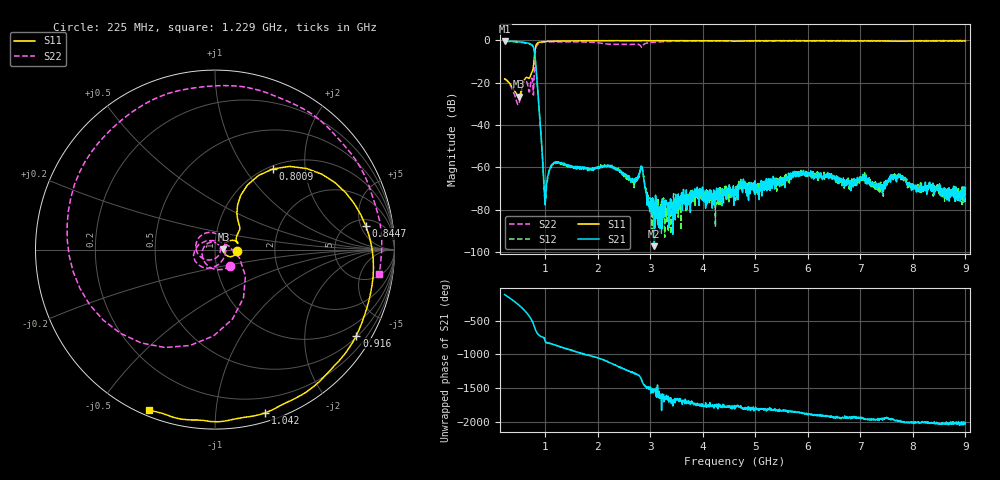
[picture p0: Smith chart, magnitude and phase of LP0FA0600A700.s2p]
!Agilent Technologies,E8358A,US41080443,A.07.50.56
!Agilent E8358A: A.07.50.56
!Date: Wednesday, August 31, 2016 09:10:34
!Correction: S11(Full 2 Port(1,2))
!S21(Full 2 Port(1,2))
!S12(Full 2 Port(1,2))
!S22(Full 2 Port(1,2))
!S2P File: Measurements: S11, S21, S12, S22:
# Hz S  dB  R 50
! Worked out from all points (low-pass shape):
!   1601 points, 225 MHz to 9 GHz, reference 50 ohm
!   highest |S21| = -0.28 dB at 225 MHz (marker M1); lowest = -97.2 dB at 3.077 GHz (marker M2)
!   |S21| within 3 dB of the highest: start of sweep to 776.3 MHz
!   lowest |S11| = -26.6 dB at 493.7 MHz (marker M3), VSWR 1.10, Z = 54.9 + j0.169 ohm
!   |S11| at or under -10 dB: start of sweep to 782.7 MHz
!   |S22| runs from -30.4 to 0.0 dB; largest |S21 - S12| = 0.021
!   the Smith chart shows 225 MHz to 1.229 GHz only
!   S11 on the Smith chart (normalised r, x): 225 MHz: 1.28, -0.01; 800.9 MHz: 1.05, +1.36; 844.7 MHz: 6.40, +6.14; 916 MHz: 0.55, -3.49; 1.042 GHz: 0.07, -1.35; 1.229 GHz: 0.02, -0.67
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2.25e8  -18.27 -2.7  -0.28 -113.7  -0.46 -113.4  -18.14 -47.5
4.937344e8  -26.58 1.9  -0.58 92.1  -0.77 92.4  -30.23 -12.7
6.034219e8  -18.56 25.7  -0.92 12.0  -1.10 12.2  -19.40 175.0
6.911719e8  -17.88 21.4  -1.39 -70.1  -1.57 -69.8  -24.24 13.4
8.008594e8  -5.14 54.3  -6.65 110.5  -6.84 110.7  -7.96 -76.0
8.447344e8  -1.41 9.0  -19.79 36.9  -19.95 36.9  -2.12 -164.1
9.160312e8  -0.71 -31.3  -43.67 -13.3  -43.90 -13.4  -1.05 130.2
1.042172e9  -0.44 -72.9  -64.58 -111.3  -66.06 -104.8  -0.72 64.6
1.228641e9  -0.30 -112.5  -57.35 -152.7  -57.68 -151.2  -0.67 -8.6
1.4535e9  -0.28 -146.6  -59.51 156.3  -59.47 152.6  -0.70 -94.3
1.689328e9  -0.15 -170.9  -59.99 98.1  -60.46 103.9  -0.72 178.9
2.001938e9  -0.11 155.8  -60.43 31.4  -60.21 29.0  -1.07 81.8
2.166469e9  -0.17 145.6  -59.76 -18.8  -59.60 -20.1  -1.60 -0.4
2.320031e9  -0.11 137.4  -60.30 -74.3  -60.35 -73.3  -1.83 -97.1
2.462625e9  -0.07 130.2  -62.80 -118.3  -62.69 -120.0  -1.80 176.3
2.621672e9  -0.15 122.8  -65.53 -177.0  -65.24 -173.1  -1.88 86.6
3.076875e9  -0.16 103.7  -97.21 -89.7  -77.84 -105.5  -0.77 -79.9
3.153656e9  -0.15 100.6  -81.99 -124.3  -81.89 -163.4  -0.67 -95.4
4.6125e9  -0.29 37.0  -71.64 16.5  -71.93 28.7  -0.12 130.4
6.076828e9  -0.21 -27.1  -64.29 -80.5  -63.36 -93.3  -0.20 41.2
7.541156e9  -0.23 -88.2  -65.21 -154.1  -65.55 -150.7  -0.11 -38.8
9e9  -0.24 -140.2  -69.65 148.7  -72.29 139.5  -0.08 -99.8
